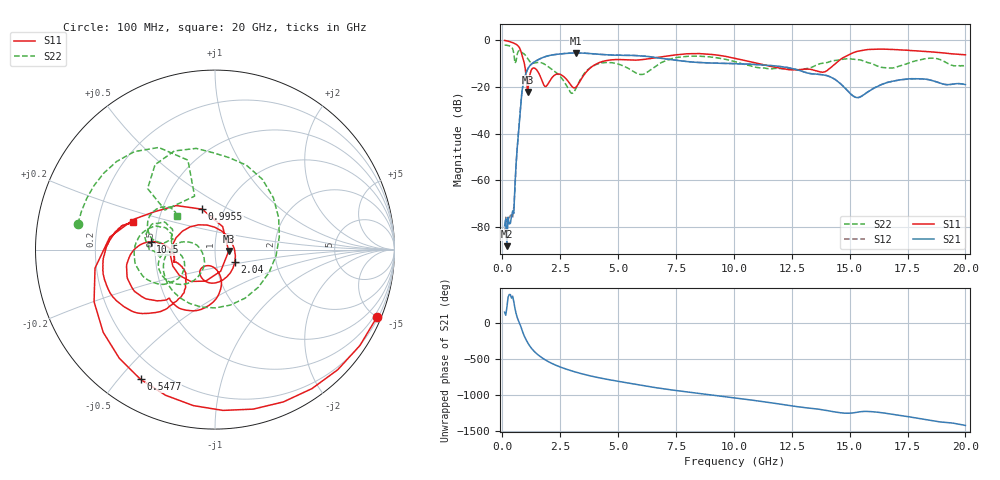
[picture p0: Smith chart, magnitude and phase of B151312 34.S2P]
!  2-Port S-parameters saved by WinCal
! VAR MeasName=S-Parameters (CALIBRATED_DATA) read from VNA (N5244A)
! VAR MeasDate=12/8/2015 5:46:17 PM
! VAR NAME=B151312 34
! VAR FILENAME=B151312 34.S2P
! VAR DATE=12/8/2015 5:46:17 PM
! VAR PHYS_PORTS=1,2
# Hz S DB R 50
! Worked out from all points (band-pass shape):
!   401 points, 100 MHz to 20 GHz, reference 50 ohm
!   highest |S21| = -5.53 dB at 3.184 GHz (marker M1); lowest = -88.2 dB at 199.5 MHz (marker M2)
!   |S21| within 3 dB of the highest: 1.529 GHz to 7.398 GHz (5.869 GHz wide, 131 % of centre)
!   lowest |S11| = -22.3 dB at 1.095 GHz (marker M3), VSWR 1.17, Z = 58.3 - j0.964 ohm
!   |S11| at or under -10 dB: 950.9 MHz to 4.112 GHz (3.161 GHz wide, 125 % of centre); 11.02 GHz to 14.4 GHz (3.382 GHz wide, 26.6 % of centre)
!   |S22| runs from -22.8 to -2.2 dB; largest |S21 - S12| = 0.0025
!   S11 on the Smith chart (normalised r, x): 100 MHz: 0.29, -4.99; 547.8 MHz: 0.12, -0.57; 995.5 MHz: 0.79, +0.38; 2.04 GHz: 1.23, -0.18; 10.5 GHz: 0.47, +0.05; 20 GHz: 0.36, +0.14
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1e8  -0.20 -22.6  -79.50 157.7  -82.93 -138.2  -2.19 169.3
1.995e8  -0.38 -44.4  -88.17 -132.9  -80.65 108.6  -2.28 158.2
3.985e8  -0.94 -87.1  -75.46 -5.8  -74.70 -1.7  -3.01 129.5
5.4775e8  -1.58 -119.8  -61.94 -150.6  -63.81 -155.6  -9.93 110.9
7.965e8  -4.58 173.2  -27.57 -39.7  -27.56 -39.7  -4.83 100.5
9.955e8  -12.53 107.7  -15.12 151.8  -15.12 151.8  -6.52 56.0
1.095e9  -22.28 -6.1  -12.49 91.3  -12.49 91.3  -8.03 26.6
1.34375e9  -11.96 -158.6  -9.64 -18.9  -9.64 -19.0  -9.94 -58.2
1.5925e9  -14.51 137.7  -8.21 -91.6  -8.21 -91.6  -9.57 -126.0
2.04025e9  -17.64 -32.5  -6.62 177.1  -6.61 177.1  -11.82 -179.1
2.5875e9  -15.16 -115.0  -5.87 100.6  -5.87 100.7  -16.61 163.7
3.1845e9  -20.12 -94.9  -5.53 38.3  -5.53 38.3  -20.69 -129.0
3.43325e9  -16.34 -78.6  -5.59 16.1  -5.58 16.1  -15.84 -121.7
4.92575e9  -8.35 -122.1  -6.49 -84.6  -6.48 -84.7  -10.09 -170.4
5.9705e9  -8.47 -133.6  -6.76 -143.1  -6.75 -143.3  -14.76 -163.7
6.7665e9  -7.36 -138.2  -7.70 175.2  -7.70 175.2  -10.25 -143.3
1.005e10  -7.82 175.4  -10.14 39.4  -10.12 39.4  -9.23 158.0
1.049775e10  -8.84 173.3  -10.26 20.4  -10.26 20.2  -10.54 156.2
1.338325e10  -12.67 -162.4  -14.49 -107.4  -14.48 -107.7  -11.60 -173.1
1.53235e10  -4.90 -142.3  -24.63 -161.7  -24.62 -161.7  -8.37 159.3
1.67165e10  -4.02 -172.1  -17.97 177.0  -17.90 176.2  -12.00 163.9
2e10  -6.34 161.4  -19.06 13.9  -19.13 13.6  -11.02 138.3
